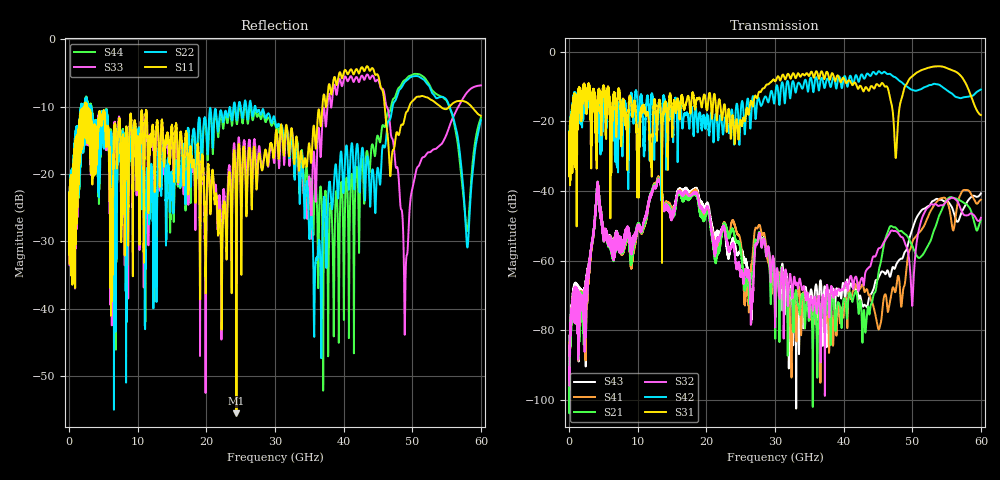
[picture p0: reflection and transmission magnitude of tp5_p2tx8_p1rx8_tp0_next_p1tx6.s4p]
! 100G CR Analysis
! File: tp5_p2tx8_p1rx8_tp0_next_p1tx6
! Description: 2m Cu Cable, OSFP, TP0-TP5
! Port Mapping
! Port1 -- P1RX8N
! Port2 -- P1TX6N
! Port3 -- P1RX8P
! Port4 -- P1TX6P
# GHz S MA R 50.00
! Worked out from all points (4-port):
!   6000 points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, 10 MHz to 60 GHz, reference 50 ohm
!   strongest paths, dB at 10 MHz, 15.01 GHz, 30.01 GHz, 45.01 GHz, 60 GHz:
!     S31: -28.2, -21.5, -8.4, -9.5, -18.2
!     S42: -27.9, -18.4, -12.9, -5.7, -10.8
!     S32: -95.9, -46.0, -78.9, -56.8, -47.7
!     S21: -93.2, -45.6, -77.1, -64.3, -48.4
!     S41: -96.8, -44.8, -67.9, -79.4, -42.5
!     S43: -90.7, -45.2, -70.0, -65.2, -40.7
!   lowest |S11| = -55.6 dB at 24.39 GHz (marker M1), VSWR 1.00, Z = 50.2 - j0.0682 ohm
!   |S11| at or under -10 dB: start of sweep to 2.216 GHz; 2.623 GHz to 36.91 GHz (34.29 GHz wide, 173 % of centre); 45.99 GHz to 49.55 GHz (3.562 GHz wide, 7.46 % of centre)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
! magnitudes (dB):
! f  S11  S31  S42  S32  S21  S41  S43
! 10 MHz  -23.9  -28.2  -27.9  -95.9  -93.2  -96.8  -90.7
! 4.16 GHz  -13.6  -14.0  -14.3  -37.3  -37.3  -37.3  -37.4
! 24.39 GHz  -55.6  -19.4  -15.1  -62.0  -54.5  -51.5  -57.7
! 35.87 GHz  -15.5  -6.1  -7.8  -70.9  -73.5  -78.0  -67.7
! 45.15 GHz  -5.8  -9.8  -5.6  -56.4  -62.6  -79.8  -64.7
! 49.04 GHz  -11.0  -9.6  -9.7  -55.5  -52.4  -64.6  -57.3
! 60 GHz  -11.4  -18.2  -10.8  -47.7  -48.4  -42.5  -40.7
